(* Logix 5000 Routine export IS7800_Job_Change; software revision 33.01 *)

VAR_GLOBAL   (* controller tags *)
   Job_ID : INT := 3;
   Job_ID_Change : BOOL;
   ONS : DINT;
END_VAR

PROGRAM MainProgram

ROUTINE IS7800_Job_Change   (* ladder *)
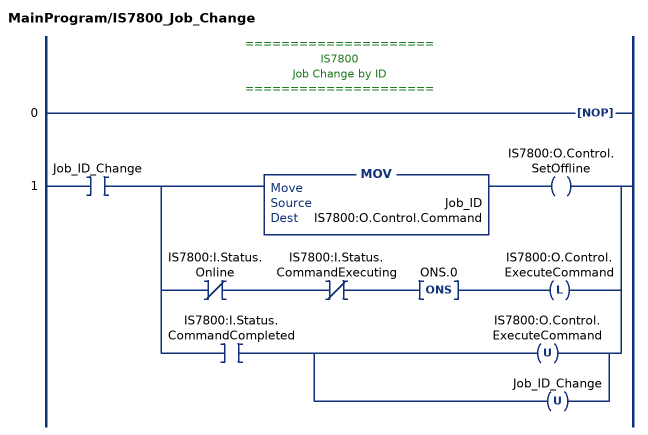
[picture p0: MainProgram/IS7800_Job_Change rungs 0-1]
   // =====================
   // IS7800
   // Job Change by ID
   // =====================
   0: NOP();
   1: XIC(Job_ID_Change)[MOV(Job_ID,IS7800:O.Control.Command) OTE(IS7800:O.Control.SetOffline) ,XIO(IS7800:I.Status.Online) XIO(IS7800:I.Status.CommandExecuting) ONS(ONS.0) OTL(IS7800:O.Control.ExecuteCommand) ,XIC(IS7800:I.Status.CommandCompleted) [OTU(IS7800:O.Control.ExecuteCommand) ,OTU(Job_ID_Change) ] ];
END_ROUTINE
END_PROGRAM
